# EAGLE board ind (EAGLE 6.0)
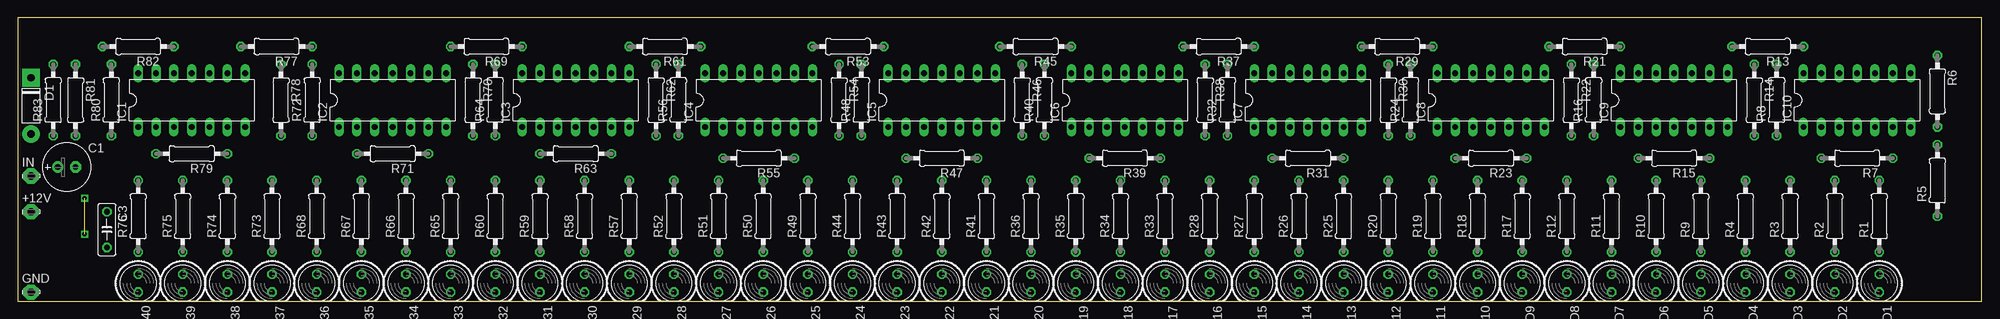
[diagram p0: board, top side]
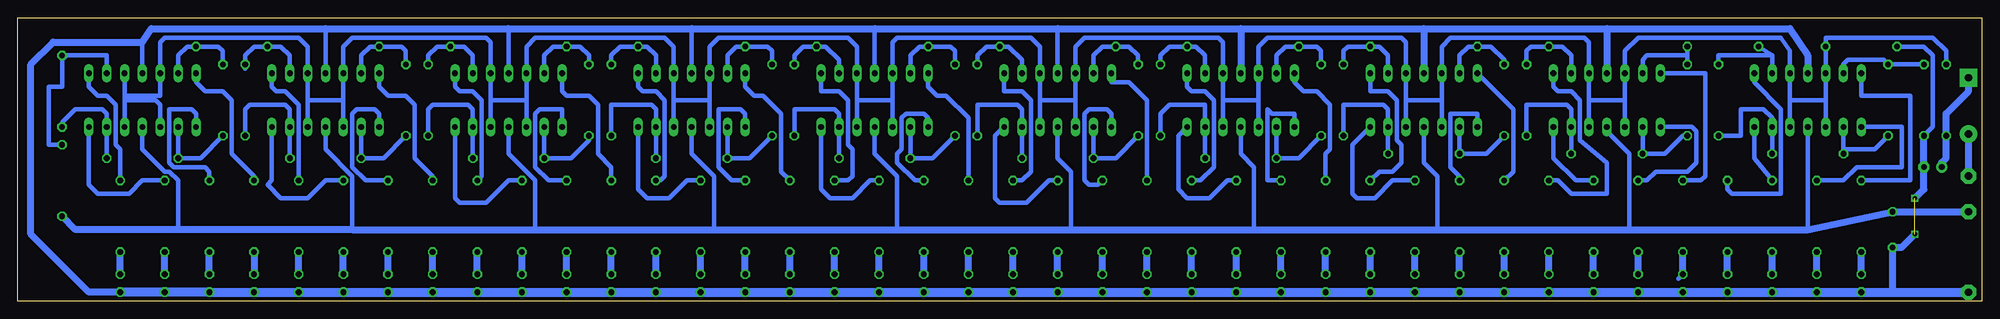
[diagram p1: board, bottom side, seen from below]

Size 279.38 x 40.31 mm. Coordinates in mm from the lower left corner, seen from the top.
Outline: 0,0 279.38,0 279.38,40.31 0,40.31 0,0
Copper layers (1*16): Top 0.035mm / dielectric 1.5mm / Bottom 0.035mm
Design rules: minimum track width 10mil, minimum drill 24mil, track to track 8mil, track to pad 8mil, pad to pad 8mil, via to via 8mil, smd to smd 8mil, copper to edge 40mil, drill to drill 8mil, minimum pad ring 10mil, minimum via ring 8mil, stop-mask expansion 4mil, vias tented up to drill 0mil, thermal gap 10mil

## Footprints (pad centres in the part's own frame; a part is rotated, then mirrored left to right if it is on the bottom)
LSP10 = drill 1.016 pad 2.159 octagon: MP 0,0
E2,5-7 = drill 0.813 pad 1.6: + -1.27,0 | drill 0.813 pad 1.6 octagon: - 1.27,0
C050-025X075 = drill 0.813 octagon: 1 -2.54,0; 2 2.54,0
DO41 = drill 1.016 pad 2.54: A 8,0 | drill 1.016 pad 2.54 square: K 0,0
DIL14 = drill 0.813 long: 1 -7.62,-3.81; 2 -5.08,-3.81; 3 -2.54,-3.81; 4 0,-3.81; 5 2.54,-3.81; 6 5.08,-3.81; 7 7.62,-3.81; 8 7.62,3.81; 9 5.08,3.81; 10 2.54,3.81; 11 0,3.81; 12 -2.54,3.81; 13 -5.08,3.81; 14 -7.62,3.81
LED5MM = drill 0.813 octagon: A -1.27,0; K 1.27,0
0207/10 = drill 0.813 octagon: 1 -5.08,0; 2 5.08,0

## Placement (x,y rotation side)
+12V  [LSP10]  1.91,12.7 0 top
C1  100u  [E2,5-7]  6.99,19.05 0 top
C3  100n  [C050-025X075]  12.7,10.16 270 top
D1  1N4148  [DO41]  1.91,31.75 270 top
GND  [LSP10]  1.91,1.27 0 top
IC1  LM324N  [DIL14]  24.77,28.57 0 top
IC2  LM324N  [DIL14]  53.34,28.57 0 top
IC3  LM324N  [DIL14]  79.38,28.57 0 top
IC4  LM324N  [DIL14]  105.41,28.57 0 top
IC5  LM324N  [DIL14]  131.44,28.57 0 top
IC6  LM324N  [DIL14]  157.48,28.57 0 top
IC7  LM324N  [DIL14]  183.51,28.57 0 top
IC8  LM324N  [DIL14]  209.55,28.57 0 top
IC9  LM324N  [DIL14]  235.59,28.57 0 top
IC10  LM324N  [DIL14]  261.62,28.57 0 top
IN  [LSP10]  1.91,17.78 0 top
LED1  [LED5MM]  264.8,2.54 270 top
LED2  [LED5MM]  258.44,2.54 270 top
LED3  [LED5MM]  252.09,2.54 270 top
LED4  [LED5MM]  245.75,2.54 270 top
LED5  [LED5MM]  239.4,2.54 270 top
LED6  [LED5MM]  233.04,2.54 270 top
LED7  [LED5MM]  226.69,2.54 270 top
LED8  [LED5MM]  220.34,2.54 270 top
LED9  [LED5MM]  214,2.54 270 top
LED10  [LED5MM]  207.65,2.54 270 top
LED11  [LED5MM]  201.29,2.54 270 top
LED12  [LED5MM]  194.94,2.54 270 top
LED13  [LED5MM]  188.59,2.54 270 top
LED14  [LED5MM]  182.25,2.54 270 top
LED15  [LED5MM]  175.9,2.54 270 top
LED16  [LED5MM]  169.54,2.54 270 top
LED17  [LED5MM]  163.19,2.54 270 top
LED18  [LED5MM]  156.84,2.54 270 top
LED19  [LED5MM]  150.5,2.54 270 top
LED20  [LED5MM]  144.15,2.54 270 top
LED21  [LED5MM]  137.79,2.54 270 top
LED22  [LED5MM]  131.44,2.54 270 top
LED23  [LED5MM]  125.09,2.54 270 top
LED24  [LED5MM]  118.75,2.54 270 top
LED25  [LED5MM]  112.39,2.54 270 top
LED26  [LED5MM]  106.05,2.54 270 top
LED27  [LED5MM]  99.69,2.54 270 top
LED28  [LED5MM]  93.34,2.54 270 top
LED29  [LED5MM]  87,2.54 270 top
LED30  [LED5MM]  80.64,2.54 270 top
LED31  [LED5MM]  74.3,2.54 270 top
LED32  [LED5MM]  67.94,2.54 270 top
LED33  [LED5MM]  61.59,2.54 270 top
LED34  [LED5MM]  55.24,2.54 270 top
LED35  [LED5MM]  48.9,2.54 270 top
LED36  [LED5MM]  42.55,2.54 270 top
LED37  [LED5MM]  36.2,2.54 270 top
LED38  [LED5MM]  29.84,2.54 270 top
LED39  [LED5MM]  23.5,2.54 270 top
LED40  [LED5MM]  17.14,2.54 270 top
R1  820R  [0207/10]  264.8,12.06 90 top
R2  820R  [0207/10]  258.44,12.06 90 top
R3  820R  [0207/10]  252.09,12.06 90 top
R4  820R  [0207/10]  245.75,12.06 90 top
R5  3M6  [0207/10]  273.05,17.14 90 top
R6  8k2  [0207/10]  273.05,29.84 270 top
R7  8k2  [0207/10]  261.62,20.32 180 top
R8  8k2  [0207/10]  250.19,28.57 90 top
R9  820R  [0207/10]  239.4,12.06 90 top
R10  820R  [0207/10]  233.04,12.06 90 top
R11  390R  [0207/10]  226.69,12.06 90 top
R12  390R  [0207/10]  220.34,12.06 90 top
R13  8k2  [0207/10]  248.92,36.2 180 top
R14  8k2  [0207/10]  247.01,28.57 270 top
R15  8k2  [0207/10]  235.59,20.32 180 top
R16  8k2  [0207/10]  224.16,28.57 90 top
R17  390R  [0207/10]  214,12.06 90 top
R18  390R  [0207/10]  207.65,12.06 90 top
R19  390R  [0207/10]  201.29,12.06 90 top
R20  390R  [0207/10]  194.94,12.06 90 top
R21  8k2  [0207/10]  222.88,36.2 180 top
R22  8k2  [0207/10]  220.98,28.57 270 top
R23  8k2  [0207/10]  209.55,20.32 180 top
R24  8k2  [0207/10]  198.12,28.57 90 top
R25  390R  [0207/10]  188.59,12.06 90 top
R26  390R  [0207/10]  182.25,12.06 90 top
R27  390R  [0207/10]  175.9,12.06 90 top
R28  390R  [0207/10]  169.54,12.06 90 top
R29  8k2  [0207/10]  196.22,36.2 180 top
R30  8k2  [0207/10]  194.94,28.57 270 top
R31  8k2  [0207/10]  183.51,20.32 180 top
R32  8k2  [0207/10]  172.09,28.57 90 top
R33  390R  [0207/10]  163.19,12.06 90 top
R34  390R  [0207/10]  156.84,12.06 90 top
R35  390R  [0207/10]  150.5,12.06 90 top
R36  390R  [0207/10]  144.15,12.06 90 top
R37  8k2  [0207/10]  170.81,36.2 180 top
R38  8k2  [0207/10]  168.91,28.57 270 top
R39  8k2  [0207/10]  157.48,20.32 180 top
R40  8k2  [0207/10]  146.05,28.57 90 top
R41  390R  [0207/10]  137.79,12.06 90 top
R42  390R  [0207/10]  131.44,12.06 90 top
R43  390R  [0207/10]  125.09,12.06 90 top
R44  390R  [0207/10]  118.75,12.06 90 top
R45  8k2  [0207/10]  144.78,36.2 180 top
R46  8k2  [0207/10]  142.88,28.57 270 top
R47  8k2  [0207/10]  131.44,20.32 180 top
R48  8k2  [0207/10]  120.02,28.57 90 top
R49  390R  [0207/10]  112.39,12.06 90 top
R50  390R  [0207/10]  106.05,12.06 90 top
R51  390R  [0207/10]  99.69,12.06 90 top
R52  390R  [0207/10]  93.34,12.06 90 top
R53  8k2  [0207/10]  118.11,36.2 180 top
R54  8k2  [0207/10]  116.84,28.57 270 top
R55  8k2  [0207/10]  105.41,20.32 180 top
R56  8k2  [0207/10]  93.98,28.57 90 top
R57  390R  [0207/10]  87,12.06 90 top
R58  390R  [0207/10]  80.64,12.06 90 top
R59  390R  [0207/10]  74.3,12.06 90 top
R60  390R  [0207/10]  67.94,12.06 90 top
R61  8k2  [0207/10]  92.08,36.2 180 top
R62  8k2  [0207/10]  90.81,28.57 270 top
R63  8k2  [0207/10]  79.38,20.95 180 top
R64  8k2  [0207/10]  67.94,28.57 90 top
R65  390R  [0207/10]  61.59,12.06 90 top
R66  390R  [0207/10]  55.24,12.06 90 top
R67  390R  [0207/10]  48.9,12.06 90 top
R68  390R  [0207/10]  42.55,12.06 90 top
R69  8k2  [0207/10]  66.67,36.2 180 top
R70  8k2  [0207/10]  64.77,28.57 270 top
R71  8k2  [0207/10]  53.34,20.95 180 top
R72  8k2  [0207/10]  41.91,28.57 90 top
R73  390R  [0207/10]  36.2,12.06 90 top
R74  390R  [0207/10]  29.84,12.06 90 top
R75  390R  [0207/10]  23.5,12.06 90 top
R76  390R  [0207/10]  17.14,12.06 90 top
R77  8k2  [0207/10]  36.83,36.2 180 top
R78  8k2  [0207/10]  37.47,28.57 270 top
R79  8k2  [0207/10]  24.77,20.95 180 top
R80  8k2  [0207/10]  13.34,28.57 90 top
R81  8k2  [0207/10]  8.26,28.57 270 top
R82  8k2  [0207/10]  17.14,36.2 180 top
R83  12R  [0207/10]  5.08,28.57 90 top

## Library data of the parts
+12V GND IN = solpad
C1 C3 R1-R83 = rcl
D1 = GM99
IC1-IC10 = linear
LED1-LED40 = led

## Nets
C1: C1.- C3.2 GND.MP IC1.11 IC2.11 IC3.11 IC4.11 IC5.11 IC6.11 IC7.11 IC8.11 IC9.11 IC10.11 LED1.K LED2.K LED3.K LED4.K LED5.K LED6.K LED7.K LED8.K LED9.K LED10.K LED11.K LED12.K LED13.K LED14.K LED15.K LED16.K LED17.K LED18.K LED19.K LED20.K LED21.K LED22.K LED23.K LED24.K LED25.K LED26.K LED27.K LED28.K LED29.K LED30.K LED31.K LED32.K LED33.K LED34.K LED35.K LED36.K LED37.K LED38.K LED39.K LED40.K R81.2 R82.2
N$1: LED1.A R1.1
N$2: LED2.A R2.1
N$3: LED3.A R3.1
N$4: IC10.14 R4.2
N$5: IC10.8 R1.2
N$6: IC10.7 R2.2
N$7: IC10.1 R3.2
N$8: LED4.A R4.1
N$9: LED17.A R33.1
N$10: IC10.9 R5.2 R6.1
N$11: IC10.6 R6.2 R7.1
N$12: IC10.2 R7.2 R8.1
N$13: IC10.13 R8.2 R13.1
N$14: LED5.A R9.1
N$15: LED6.A R10.1
N$16: LED7.A R11.1
N$17: IC9.14 R12.2
N$18: IC9.8 R9.2
N$19: IC9.7 R10.2
N$20: IC9.1 R11.2
N$21: LED8.A R12.1
N$22: LED18.A R34.1
N$23: IC9.9 R13.2 R14.1
N$24: IC9.6 R14.2 R15.1
N$25: IC9.2 R15.2 R16.1
N$26: IC9.13 R16.2 R21.1
N$27: LED9.A R17.1
N$28: LED10.A R18.1
N$29: LED11.A R19.1
N$30: IC8.14 R20.2
N$31: IC8.8 R17.2
N$32: IC8.7 R18.2
N$33: IC8.1 R19.2
N$34: LED12.A R20.1
N$35: IC8.9 R21.2 R22.1
N$36: IC8.6 R22.2 R23.1
N$37: IC8.2 R23.2 R24.1
N$38: IC8.13 R24.2 R29.1
N$39: LED13.A R25.1
N$40: LED14.A R26.1
N$41: LED15.A R27.1
N$42: IC7.14 R28.2
N$43: IC7.8 R25.2
N$44: IC7.7 R26.2
N$45: IC7.1 R27.2
N$46: LED16.A R28.1
N$47: D1.A IN.MP
N$48: IC7.9 R29.2 R30.1
N$49: IC7.6 R30.2 R31.1
N$50: IC7.2 R31.2 R32.1
N$51: IC7.13 R32.2 R37.1
N$52: LED19.A R35.1
N$53: IC6.14 R36.2
N$54: IC6.8 R33.2
N$55: IC6.7 R34.2
N$56: IC6.1 R35.2
N$57: LED20.A R36.1
N$58: IC6.9 R37.2 R38.1
N$59: IC6.6 R38.2 R39.1
N$60: IC6.2 R39.2 R40.1
N$61: IC6.13 R40.2 R45.1
N$62: LED21.A R41.1
N$63: LED22.A R42.1
N$64: LED23.A R43.1
N$65: IC5.14 R44.2
N$66: IC5.8 R41.2
N$67: IC5.7 R42.2
N$68: IC5.1 R43.2
N$69: LED24.A R44.1
N$70: IC5.9 R45.2 R46.1
N$71: IC5.6 R46.2 R47.1
N$72: IC5.2 R47.2 R48.1
N$73: IC5.13 R48.2 R53.1
N$74: LED25.A R49.1
N$75: LED26.A R50.1
N$76: LED27.A R51.1
N$77: IC4.14 R52.2
N$78: IC4.8 R49.2
N$79: IC4.7 R50.2
N$80: IC4.1 R51.2
N$81: LED28.A R52.1
N$82: IC4.9 R53.2 R54.1
N$83: IC4.6 R54.2 R55.1
N$84: IC4.2 R55.2 R56.1
N$85: IC4.13 R56.2 R61.1
N$86: LED29.A R57.1
N$87: LED30.A R58.1
N$88: LED31.A R59.1
N$89: IC3.14 R60.2
N$90: IC3.8 R57.2
N$91: IC3.7 R58.2
N$92: IC3.1 R59.2
N$93: LED32.A R60.1
N$95: IC3.9 R61.2 R62.1
N$96: IC3.6 R62.2 R63.1
N$97: IC3.2 R63.2 R64.1
N$98: IC3.13 R64.2 R69.1
N$99: LED33.A R65.1
N$100: LED34.A R66.1
N$101: LED35.A R67.1
N$102: IC2.14 R68.2
N$103: IC2.8 R65.2
N$104: IC2.7 R66.2
N$105: IC2.1 R67.2
N$106: LED36.A R68.1
N$107: IC2.9 R69.2 R70.1
N$108: IC2.6 R70.2 R71.1
N$109: IC2.2 R71.2 R72.1
N$110: IC2.13 R72.2 R77.1
N$111: LED37.A R73.1
N$112: LED38.A R74.1
N$113: LED39.A R75.1
N$114: IC1.14 R76.2
N$115: IC1.8 R73.2
N$116: IC1.7 R74.2
N$117: IC1.1 R75.2
N$118: LED40.A R76.1
N$119: +12V.MP C3.1 IC1.4 IC2.4 IC3.4 IC4.4 IC5.4 IC6.4 IC7.4 IC8.4 IC9.4 IC10.4 R5.1
N$120: IC1.9 R77.2 R78.1
N$121: IC1.6 R78.2 R79.1
N$122: IC1.2 R79.2 R80.1
N$123: IC1.13 R80.2 R81.1
N$124: IC1.3 IC1.5 IC1.10 IC1.12 IC2.3 IC2.5 IC2.10 IC2.12 IC3.3 IC3.5 IC3.10 IC3.12 IC4.3 IC4.5 IC4.10 IC4.12 IC5.3 IC5.5 IC5.10 IC5.12 IC6.3 IC6.5 IC6.10 IC6.12 IC7.3 IC7.5 IC7.10 IC7.12 IC8.3 IC8.5 IC8.10 IC8.12 IC9.3 IC9.5 IC9.10 IC9.12 IC10.3 IC10.5 IC10.10 IC10.12 R82.1 R83.2
N$125: C1.+ D1.K R83.1

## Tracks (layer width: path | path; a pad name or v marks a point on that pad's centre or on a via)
C1  (via drill 0.6)  (1 unrouted)
  Bottom 0.61: LED15.K 176.53,1.27 | LED5.K 240.03,1.27 | 261.62,36.83 IC10.11 | 131.44,38.73 IC5.11 | 157.48,38.73 IC6.11 | 183.51,38.73 IC7.11 | 209.55,38.73 IC8.11 | 235.59,38.73 IC9.11 | R82.2 8.26,36.2 6.99,34.92 6.99,24.77 R81.2
  Bottom 1.016: 105.41,38.73 131.44,38.73 157.48,38.73 183.51,38.73 209.55,38.73 235.59,38.73 260.35,38.73 261.62,36.83 274.32,36.83 277.5,33.66 277.5,9.53 269.24,1.27 LED1.K | 105.41,38.73 79.38,38.73 | 79.38,38.73 53.34,38.73 | 53.34,38.73 27.3,38.73 24.77,34.92 IC1.11 | 53.34,38.73 IC2.11 | 79.38,38.73 IC3.11 | 105.41,38.73 IC4.11 | 12.7,1.27 C3.2 11.43,7.62 v9.53,9.53 | R81.2 C1.- 8.26,15.88 v9.53,14.61
  Bottom 1.27: GND.MP 12.7,1.27 LED40.K LED39.K LED38.K LED37.K LED36.K LED35.K LED34.K LED33.K LED32.K LED31.K LED30.K LED29.K LED28.K LED27.K LED26.K LED25.K LED24.K LED23.K LED22.K LED21.K LED20.K LED19.K LED18.K LED17.K LED16.K LED15.K LED14.K LED13.K LED12.K LED11.K LED10.K LED9.K LED8.K LED7.K LED6.K LED5.K LED4.K LED3.K LED2.K LED1.K
N$1
  Bottom 1.016: LED1.A R1.1
N$2
  Bottom 1.016: LED2.A R2.1
N$3
  Bottom 1.016: LED3.A R3.1
N$4
  Bottom 0.61: R4.2 245.75,17.78 248.92,20.95 248.92,28.57 250.19,29.84 252.73,29.84 254,31.11 IC10.14
N$5
  Bottom 0.61: R1.2 264.8,21.59 265.43,22.23 265.43,27.94 266.7,29.21 267.97,29.21 269.24,30.48 IC10.8
N$6
  Bottom 0.61: R2.2 261.62,17.14 263.52,15.24 267.97,15.24 269.24,16.51 IC10.7
N$7
  Bottom 0.61: IC10.1 254,26.67 254.63,27.3 257.81,27.3 257.81,19.68 257.18,19.05 252.73,19.05 252.09,18.41 R3.2
N$8
  Bottom 1.016: R4.1 LED4.A
N$9
  Bottom 1.016: LED17.A R33.1
N$10
  Bottom 0.61: IC10.9 266.7,34.92 272.42,34.92 273.05,34.29 R6.1 273.05,30.48 274.95,30.48 274.95,22.23 R5.2
N$11
  Bottom 0.61: R7.1 IC10.6 266.7,26.67 267.33,27.3 271.14,27.3 273.05,25.4 R6.2
N$12
  Bottom 0.61: IC10.2 R7.2 253.37,20.32 R8.1
N$13
  Bottom 0.61: IC10.13 256.54,34.92 255.27,36.2 R13.1 250.82,36.2 250.19,35.56 R8.2
N$14
  Bottom 1.016: LED5.A R9.1
N$15
  Bottom 1.016: LED6.A R10.1
N$16
  Bottom 1.016: LED7.A R11.1
N$17
  Bottom 0.61: R12.2 220.34,17.78 222.88,20.32 222.88,27.94 224.16,29.21 226.69,29.21 227.97,30.48 IC9.14
N$18
  Bottom 0.61: R9.2 239.4,27.94 241.3,29.84 242.57,29.84 243.21,30.48 IC9.8
N$19
  Bottom 0.61: R10.2 235.59,17.14 238.12,14.61 241.94,14.61 243.84,16.51 243.21,17.14 IC9.7
N$20
  Bottom 0.61: R11.2 229.87,17.14 231.78,19.05 231.78,26.67 231.14,27.3 228.6,27.3 227.97,26.67 IC9.1
N$21
  Bottom 1.016: LED8.A R12.1
N$22
  Bottom 1.016: LED18.A R34.1
N$23
  Bottom 0.61: 247.01,33.02 R14.1 247.01,34.92 245.75,36.2 R13.2 241.94,36.2 240.66,34.92 IC9.9
N$24
  Bottom 0.61: R15.1 IC9.6 240.66,27.3 241.3,27.94 246.38,27.94 247.01,27.3 R14.2
N$25
  Bottom 0.61: IC9.2 R15.2 227.33,20.32 R16.1
N$26
  Bottom 0.61: IC9.13 230.5,34.92 229.24,36.2 R21.1 224.79,36.2 224.16,35.56 R16.2
N$27
  Bottom 1.016: LED9.A R17.1
N$28
  Bottom 1.016: LED10.A R18.1
N$29
  Bottom 1.016: LED11.A R19.1
N$30
  Bottom 0.61: R20.2 194.94,19.05 196.85,20.95 196.85,27.94 198.12,29.21 201.29,29.21 201.93,29.84 IC8.14
N$31
  Bottom 0.61: R17.2 213.36,17.78 213.36,28.57 214.63,29.84 216.53,29.84 217.17,30.48 IC8.8
N$32
  Bottom 0.61: R18.2 209.55,17.14 212.72,13.97 216.53,13.97 217.17,14.61 IC8.7
N$33
  Bottom 0.61: R19.2 203.84,17.14 205.74,19.05 205.74,26.67 205.1,27.3 201.93,27.3 IC8.1
N$34
  Bottom 1.016: LED12.A R20.1
N$35
  Bottom 0.61: IC8.9 214.63,34.92 215.9,36.2 R21.2 219.71,36.2 220.98,34.92 R22.1
N$36
  Bottom 0.61: R22.2 220.98,27.3 220.34,27.94 215.26,27.94 214.63,27.3 IC8.6 R23.1
N$37
  Bottom 0.61: IC8.2 R23.2 200.66,20.32 198.12,22.86 R24.1
N$38
  Bottom 0.61: IC8.13 204.47,34.92 203.2,36.2 R29.1 199.39,36.2 198.12,34.92 R24.2
N$39
  Bottom 1.016: LED13.A R25.1
N$40
  Bottom 1.016: LED14.A R26.1
N$41
  Bottom 1.016: LED15.A R27.1
N$42
  Bottom 0.61: IC7.14 175.9,30.48 174.62,29.21 173.35,29.21 170.81,26.67 170.81,18.41 R28.2
N$43
  Bottom 0.61: R25.2 187.96,17.14 187.32,17.78 187.32,28.57 188.59,29.84 190.5,29.84 191.13,30.48 IC7.8
N$44
  Bottom 0.61: R26.2 184.15,17.14 186.69,14.61 189.87,14.61 191.13,15.88 IC7.7
N$45
  Bottom 0.61: R27.2 177.8,17.14 179.71,19.05 179.71,27.3 176.53,27.3 175.9,26.67 IC7.1
N$46
  Bottom 1.016: LED16.A R28.1
N$47
  Bottom 1.016: IN.MP D1.A
N$48
  Bottom 0.61: R30.1 194.94,34.92 193.68,36.2 R29.2 189.87,36.2 188.59,34.92 IC7.9
N$49
  Bottom 0.61: R31.1 IC7.6 188.59,27.3 189.23,27.94 194.94,27.94 R30.2
N$50
  Bottom 0.61: IC7.2 R31.2 175.26,20.32 R32.1
N$51
  Bottom 0.61: IC7.13 178.44,34.92 177.16,36.2 R37.1 172.72,36.2 172.09,35.56 R32.2
N$52
  Bottom 1.016: LED19.A R35.1
N$53
  Bottom 0.61: R36.2 144.15,26.04 147.32,29.21 148.59,29.21 149.86,30.48 IC6.14
N$54
  Bottom 0.61: R33.2 161.29,17.14 160.66,17.78 160.66,21.59 161.29,22.23 161.29,28.57 162.56,29.84 165.1,29.84 IC6.8
N$55
  Bottom 0.61: R34.2 158.12,17.14 160.66,14.61 163.83,14.61 165.1,15.88 IC6.7
N$56
  Bottom 0.61: R35.2 151.76,17.14 154.31,19.68 154.31,20.95 153.67,21.59 153.67,26.04 153.03,26.67 150.5,26.67 149.86,26.04 IC6.1
N$57
  Bottom 1.016: LED20.A R36.1
N$58
  Bottom 0.61: IC6.9 162.56,34.29 164.47,36.2 R37.2 167.64,36.2 168.91,34.92 R38.1
N$59
  Bottom 0.61: R39.1 IC6.6 162.56,26.67 163.19,27.3 168.91,27.3 R38.2
N$60
  Bottom 0.61: R40.1 149.22,20.32 R39.2 IC6.2
N$61
  Bottom 0.61: R40.2 146.05,35.56 146.69,36.2 R45.1 151.13,36.2 152.4,34.92 IC6.13
N$62
  Bottom 1.016: LED21.A R41.1
N$63
  Bottom 1.016: LED22.A R42.1
N$64
  Bottom 1.016: LED23.A R43.1
N$65
  Bottom 0.61: R44.2 118.75,28.57 121.28,31.11 123.83,31.11 IC5.14
N$66
  Bottom 0.61: R41.2 136.53,17.14 135.25,18.41 135.25,28.57 136.53,29.84 139.06,29.84 IC5.8
N$67
  Bottom 0.61: R42.2 132.72,17.14 135.89,13.97 139.7,13.97 140.34,14.61 140.34,23.5 IC5.7
N$68
  Bottom 0.61: IC5.1 123.83,26.67 124.46,27.3 127,27.3 127.64,26.67 127.64,17.14 127,16.51 125.73,16.51 R43.2
N$69
  Bottom 1.016: LED24.A R44.1
N$70
  Bottom 0.61: IC5.9 136.53,34.29 138.43,36.2 R45.2 141.6,36.2 142.88,34.92 R46.1
N$71
  Bottom 0.61: R46.2 142.88,27.94 137.16,27.94 136.53,27.3 IC5.6 R47.1
N$72
  Bottom 0.61: IC5.2 R47.2 123.19,20.32 R48.1
N$73
  Bottom 0.61: R48.2 120.02,34.92 121.28,36.2 R53.1 125.09,36.2 126.36,34.92 IC5.13
N$74
  Bottom 1.016: LED25.A R49.1
N$75
  Bottom 1.016: LED26.A R50.1
N$76
  Bottom 1.016: LED27.A R51.1
N$77
  Bottom 0.61: R52.2 93.34,20.95 92.71,21.59 92.71,27.94 94.61,29.84 96.52,29.84 97.79,31.11 IC4.14
N$78
  Bottom 0.61: R49.2 111.12,17.14 109.22,19.05 109.22,28.57 110.49,29.84 112.39,29.84 113.03,30.48 IC4.8
N$79
  Bottom 0.61: R50.2 107.31,17.14 109.86,14.61 113.03,14.61 114.3,15.88 114.3,23.5 IC4.7
N$80
  Bottom 0.61: IC4.1 97.79,26.67 100.97,26.67 101.6,27.3 101.6,17.14 R51.2
N$81
  Bottom 1.016: LED28.A R52.1
N$82
  Bottom 0.61: IC4.9 110.49,34.92 111.76,36.2 R53.2 115.57,36.2 116.84,34.92 R54.1
N$83
  Bottom 0.61: R55.1 IC4.6 110.49,27.94 115.57,27.94 116.84,26.67 R54.2
N$84
  Bottom 0.61: IC4.2 R55.2 97.16,20.32 R56.1
N$85
  Bottom 0.61: R56.2 93.98,35.56 94.61,36.2 R61.1 99.06,36.2 100.33,34.92 IC4.13
N$86
  Bottom 1.016: LED29.A R57.1
N$87
  Bottom 1.016: LED30.A R58.1
N$88
  Bottom 1.016: LED31.A R59.1
N$89
  Bottom 0.61: IC3.14 66.67,27.3 66.67,18.41 R60.2
N$90
  Bottom 0.61: R57.2 85.72,18.41 83.82,18.41 82.55,19.68 82.55,22.23 83.19,22.86 83.19,28.57 84.45,29.84 87,29.84 IC3.8
N$91
  Bottom 0.61: R58.2 83.82,17.14 86.36,14.61 88.9,14.61 89.53,15.24 89.53,22.23 IC3.7
N$92
  Bottom 0.61: R59.2 74.3,17.78 75.56,19.05 75.56,26.67 71.75,26.67 IC3.1
N$93
  Bottom 1.016: LED32.A R60.1
N$95
  Bottom 0.61: 84.45,31.75 IC3.9 84.45,34.92 85.72,36.2 R61.2 90.17,36.2 90.81,35.56 R62.1
N$96
  Bottom 0.61: R63.1 IC3.6 84.45,27.3 85.09,27.94 90.81,27.94 R62.2
N$97
  Bottom 0.61: 74.3,21.59 R63.2 | 74.3,21.59 IC3.2 | R64.1 70.48,20.95 73.66,20.95 74.3,21.59
N$98
  Bottom 0.61: IC3.13 74.3,34.92 73.03,36.2 R69.1 69.85,36.2 67.94,34.29 R64.2
N$99
  Bottom 1.016: LED33.A R65.1
N$100
  Bottom 1.016: LED34.A R66.1
N$101
  Bottom 1.016: LED35.A R67.1
N$102
  Bottom 0.61: R68.2 40.01,17.14 39.37,17.78 39.37,32.38 IC2.14
N$103
  Bottom 0.61: R65.2 60.33,17.14 58.42,15.24 53.34,15.24 53.34,19.68 57.15,22.86 57.15,28.57 58.42,29.84 60.33,29.84 60.96,30.48 IC2.8
N$104
  Bottom 0.61: R66.2 57.78,17.14 60.96,20.32 IC2.7
N$105
  Bottom 0.61: R67.2 47.62,17.14 46.35,18.41 41.91,18.41 40.64,19.68 40.64,24.13 41.27,24.77 IC2.1
N$106
  Bottom 0.61: 43.18,3.17 LED36.A
  Bottom 1.016: LED36.A R68.1
N$107
  Bottom 0.61: IC2.9 58.42,34.92 59.69,36.2 R69.2 64.14,36.2 64.77,35.56 R70.1
N$108
  Bottom 0.61: R71.1 IC2.6 58.42,27.3 59.05,27.94 64.77,27.94 R70.2
N$109
  Bottom 0.61: IC2.2 R71.2 45.09,20.95 42.55,23.5 R72.1
N$110
  Bottom 0.61: 41.91,34.92 R77.1 | R72.2 41.91,34.92 | 41.91,34.92 47.62,34.92 48.26,34.29 IC2.13
N$111
  Bottom 1.016: LED37.A R73.1
N$112
  Bottom 1.016: LED38.A R74.1
N$113
  Bottom 1.016: LED39.A R75.1
N$114
  Bottom 0.61: R76.2 10.16,17.14 10.16,29.21 17.14,29.21 IC1.14
N$115
  Bottom 0.61: IC1.8 32.38,31.11 28.57,27.3 28.57,15.24 35.56,15.24 36.2,15.88 R73.2
N$116
  Bottom 0.61: R74.2 32.38,20.32 IC1.7
N$117
  Bottom 0.61: R75.2 19.68,17.14 17.78,19.05 11.43,19.05 11.43,24.77 IC1.1
N$118
  Bottom 1.016: LED40.A R76.1
N$119
  Bottom 0.61: IC10.4 261.62,21.59 258.44,18.41 257.81,18.41 256.54,17.14 256.54,10.16 | 24.77,10.16 IC1.4 | IC9.4 235.59,21.59 231.78,17.78 231.78,10.16 | IC8.4 209.55,20.95 205.74,17.14 205.74,10.16 | IC7.4 183.51,20.95 180.34,17.78 180.34,10.16 | IC6.4 157.48,20.95 154.31,17.78 154.31,10.16 | IC5.4 131.44,20.32 129.54,18.41 129.54,10.16 | IC4.4 105.41,20.95 103.5,19.05 103.5,10.16 | IC3.4 79.38,19.68 77.47,17.78 77.47,10.16 | IC2.4 53.34,24.13 50.16,20.95 50.16,10.16
  Bottom 1.016: R5.1 271.14,10.16 256.54,10.16 231.78,10.16 205.74,10.16 180.34,10.16 154.31,10.16 129.54,10.16 103.5,10.16 77.47,10.16 50.16,10.16 24.77,10.16 C3.1 +12V.MP
N$120
  Bottom 0.61: IC1.9 29.84,34.92 | 29.84,34.92 R77.2 | R78.1 37.47,34.92 29.84,34.92
N$121
  Bottom 0.61: R79.1 IC1.6 29.84,26.04 31.11,27.3 34.29,27.3 34.29,23.5 R78.2
N$122
  Bottom 0.61: R80.1 15.24,21.59 19.68,21.59 | R79.2 19.68,21.59 | 19.68,21.59 IC1.2
N$123
  Bottom 0.61: R81.1 R80.2 13.97,34.29 19.05,34.29 19.68,33.66 IC1.13
N$124
  Bottom 0.61: 27.3,28.57 IC1.5 27.3,24.13 | 27.3,28.57 IC1.10 27.3,35.56 28.57,37.47 48.9,37.47 50.8,35.56 IC2.12 50.8,28.57 | 22.23,28.57 IC1.3 | 22.23,28.57 IC1.12 | 27.3,28.57 22.23,28.57 | IC1.12 R82.1 | 160.02,28.57 IC6.5 | 133.99,28.57 IC5.5 | 81.92,28.57 IC3.5 | 107.95,28.57 IC4.5 | 55.88,28.57 IC2.5 55.88,24.13 | 186.06,28.57 IC7.5 | 212.09,28.57 IC8.5 | 238.12,28.57 IC9.5 | 238.12,28.57 IC9.10 238.12,36.2 239.4,37.47 258.44,37.47 259.08,36.83 IC10.12 259.08,29.21 264.16,29.21 | 264.16,29.21 264.16,28.57 | 264.16,29.21 IC10.10 | 264.16,28.57 IC10.5 | 264.16,28.57 259.71,28.57 259.08,27.94 IC10.3 | 212.09,28.57 IC8.10 212.09,36.83 212.72,37.47 231.78,37.47 233.04,36.2 IC9.12 233.04,28.57 | 212.09,28.57 207.01,28.57 | 207.01,28.57 IC8.12 207.01,36.2 205.74,37.47 187.32,37.47 186.06,36.2 IC7.10 186.06,28.57 | 233.04,28.57 238.12,28.57 | IC9.3 233.04,28.57 | 207.01,28.57 IC8.3 | 180.97,28.57 IC7.3 | 154.94,28.57 IC6.3 | 154.94,28.57 IC6.12 154.94,36.83 154.31,37.47 135.25,37.47 133.99,36.2 IC5.10 133.99,28.57 | 160.02,28.57 IC6.10 160.02,36.2 161.29,37.47 179.71,37.47 180.97,36.2 IC7.12 180.97,28.57 | 160.02,28.57 154.94,28.57 | 133.99,28.57 128.91,28.57 | 128.91,28.57 IC5.12 128.91,36.2 127.64,37.47 108.58,37.47 107.95,36.83 IC4.10 107.95,28.57 | 128.91,28.57 IC5.3 | 107.95,28.57 102.87,28.57 | 102.87,28.57 IC4.12 102.87,36.2 101.6,37.47 82.55,37.47 81.92,36.83 IC3.10 81.92,28.57 | 102.87,28.57 IC4.3 | 81.92,28.57 76.83,28.57 IC3.12 | IC3.12 IC3.3 | 55.88,28.57 IC2.10 55.88,36.83 56.52,37.47 75.56,37.47 76.83,36.2 IC3.12 | 55.88,28.57 50.8,28.57 | 50.8,28.57 IC2.3 50.8,24.13 | 186.06,28.57 180.97,28.57 | IC1.12 22.23,37.47 6.99,37.47 5.08,35.56 R83.2
N$125
  Bottom 1.016: C1.+ 5.71,19.68 5.08,20.32 R83.1 5.08,26.67 1.91,29.84 D1.K

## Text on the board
Top: 25x Green LED | 9x Yellow LED | 6x Red LED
